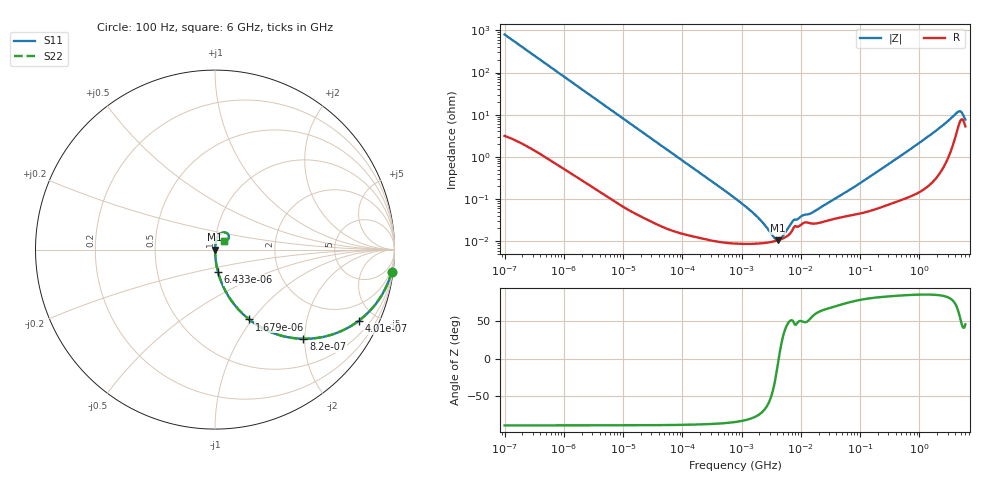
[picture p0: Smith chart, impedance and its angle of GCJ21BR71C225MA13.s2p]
!Murata Part Number: GCJ21BR71C225MA13
!These Parameters are Measured in Series Mode Connection
!Data Generated on Mar 13, 2026
!  o--ll--o
!Port1  Port2
!  o------o
!Operation Temp=25[degC], DC Bias Voltage=0[V]
!Freq. Start=100[Hz] Stop=6[GHz] 401[Steps]
# Hz S RI R 50
!Freq.(Hz) S11(Real) S11(Imag) S21(Real) S21(Imag) S12(Real) S12(Imag) S22(Real) S22(Imag)
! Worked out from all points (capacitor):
!   401 points, 100 Hz to 6 GHz, reference 50 ohm
!   read as one part in series: C = 1.98 uF near 109 Hz
!   lowest |Z| = 10.5 mohm at 4.06 MHz (marker M1)
!   series resonance near 4.238 MHz, so ESL is about 710 pH
!   S11 on the Smith chart (normalised r, x): 100 Hz: 1, -16; 401 Hz: 1.02, -4.02; 820 Hz: 1.01, -1.97; 1.679 kHz: 1.01, -0.96; 6.433 kHz: 1.00, -0.25; 6 GHz: 1.11, +0.11
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100  0.9842 -0.1228  0.0158 0.1228  0.0158 0.1228  0.9842 -0.1228
224  0.9268 -0.2579  0.0732 0.2579  0.0732 0.2579  0.9268 -0.2579
401  0.8001 -0.3971  0.1999 0.3971  0.1999 0.3971  0.8001 -0.3971
820  0.4921 -0.4968  0.5079 0.4968  0.5079 0.4968  0.4921 -0.4968
1679  0.1903 -0.3892  0.8097 0.3892  0.8097 0.3892  0.1903 -0.3892
2008  0.1417 -0.3454  0.8583 0.3454  0.8583 0.3454  0.1417 -0.3454
3287  0.059 -0.2321  0.941 0.2321  0.941 0.2321  0.059 -0.2321
6433  0.0167 -0.1244  0.9833 0.1244  0.9833 0.1244  0.0167 -0.1244
40335  0.000652 -0.0203  0.9993 0.0203  0.9993 0.0203  0.000652 -0.0203
774597  8.86e-05 -0.00104  0.9999 0.00104  0.9999 0.00104  8.86e-05 -0.00104
1813585  8.75e-05 -0.000376  0.9999 0.000376  0.9999 0.000376  8.75e-05 -0.000376
3549919  9.89e-05 -7.03e-05  0.9999 7.03e-05  0.9999 7.03e-05  9.89e-05 -7.03e-05
4060267  0.000104 -1.69e-05  0.9999 1.69e-05  0.9999 1.69e-05  0.000104 -1.69e-05
4856642  0.000114 5.44e-05  0.9999 -5.44e-05  0.9999 -5.44e-05  0.000114 5.44e-05
7599586  0.000211 0.00024  0.9998 -0.00024  0.9998 -0.00024  0.000211 0.00024
1.087309e7  0.000265 0.000313  0.9997 -0.000313  0.9997 -0.000313  0.000265 0.000313
1.555665e7  0.000261 0.000395  0.9997 -0.000395  0.9997 -0.000395  0.000261 0.000395
3.124326e8  0.000793 0.00689  0.9992 -0.00689  0.9992 -0.00689  0.000793 0.00689
1.565993e9  0.00342 0.0336  0.9966 -0.0336  0.9966 -0.0336  0.00342 0.0336
4.385646e9  0.0512 0.0959  0.9488 -0.0959  0.9488 -0.0959  0.0512 0.0959
5.016141e9  0.0766 0.0796  0.9234 -0.0796  0.9234 -0.0796  0.0766 0.0796
6e9  0.0529 0.0496  0.9471 -0.0496  0.9471 -0.0496  0.0529 0.0496
